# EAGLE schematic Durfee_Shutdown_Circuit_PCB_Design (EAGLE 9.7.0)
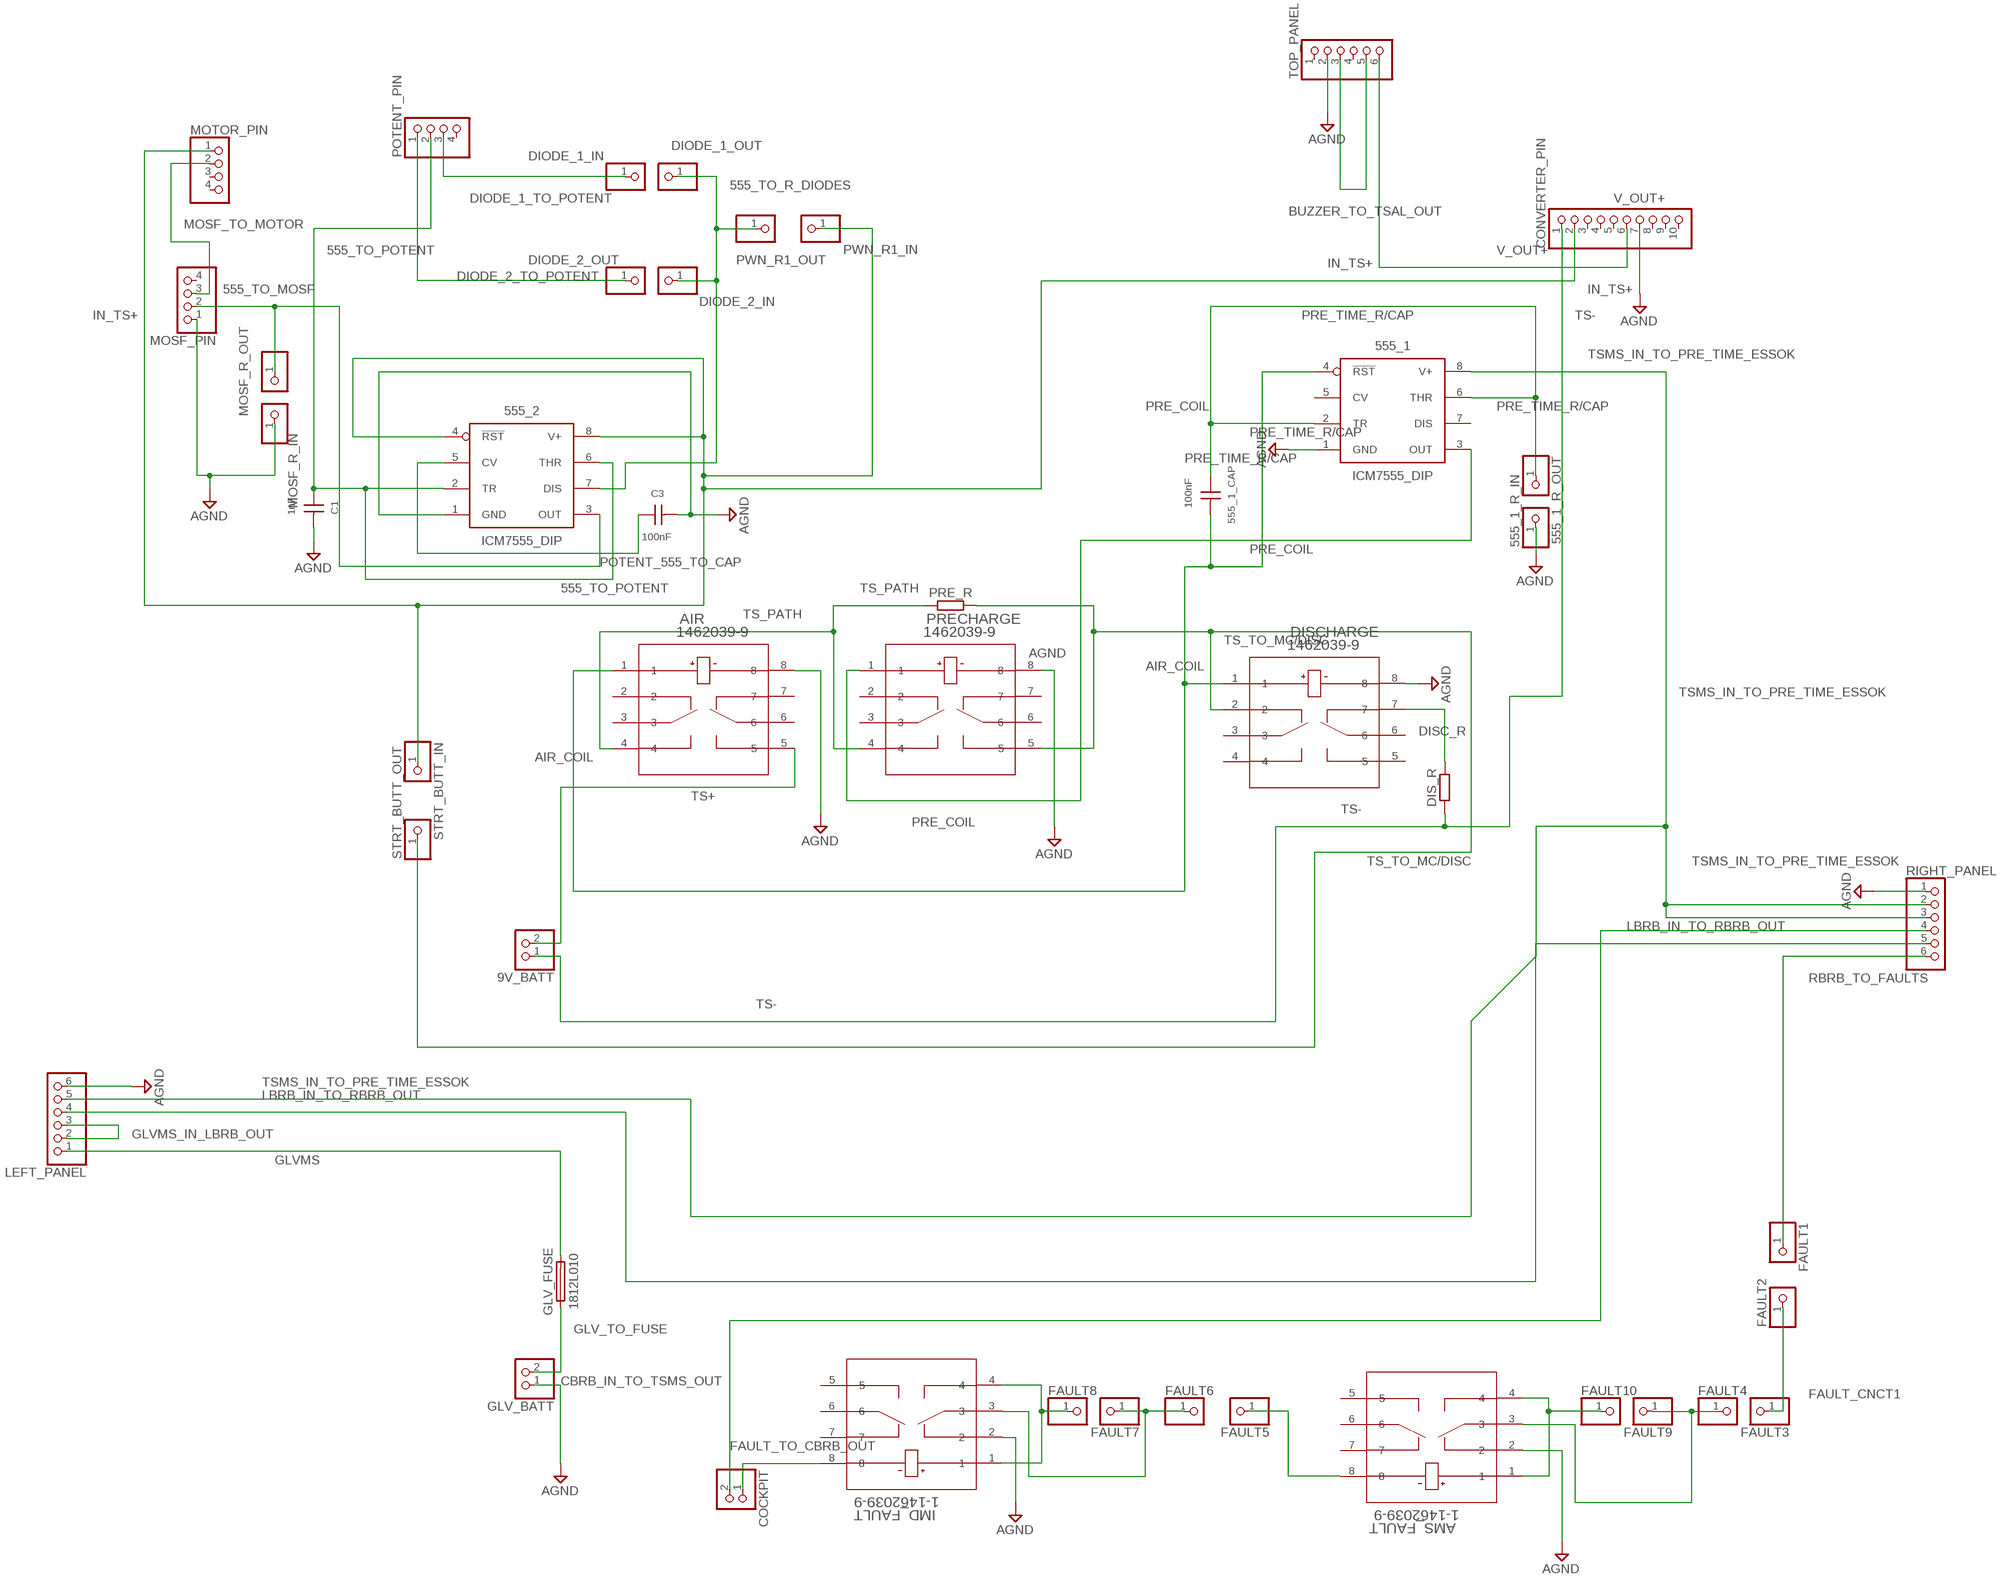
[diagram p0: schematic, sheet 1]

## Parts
9V_BATT  PINHD-1X2  [1X02]
555_1  ICM7555_DIP  [DIP826W53P254L959H508Q8B]
555_1_CAP  100nF  WCAP-CSGP_0603_885012206071_25V(DC)_R  [WCAP-CSGP_0603_R]
555_1_R_IN  PINHD-1X1  [1X01]
555_1_R_OUT  PINHD-1X1  [1X01]
555_2  ICM7555_DIP  [DIP826W53P254L959H508Q8B]
AIR  1462039-9  [RELAY8_SMTGUL]
AMS_FAULT  1-1462039-9  [RELAY8_SMTGUL]
C1  1nF  WCAP-CSGP_0402_885012205044_25V(DC)  [WCAP-CSGP_0402]
C3  100nF  WCAP-CSGP_0603_885012206071_25V(DC)_R  [WCAP-CSGP_0603_R]
COCKPIT  PINHD-1X2  [1X02]
CONVERTER_PIN  PINHD-1X10  [1X10]
DIODE_1_IN  PINHD-1X1  [1X01]
DIODE_1_OUT  PINHD-1X1  [1X01]
DIODE_2_IN  PINHD-1X1  [1X01]
DIODE_2_OUT  PINHD-1X1  [1X01]
DIS_R  R_AXIAL-7.2MM-PITCH  [RESAD724W46L381D178B]
DISCHARGE  1462039-9  [RELAY8_SMTGUL]
FAULT1  PINHD-1X1  [1X01]
FAULT2  PINHD-1X1  [1X01]
FAULT3  PINHD-1X1  [1X01]
FAULT4  PINHD-1X1  [1X01]
FAULT5  PINHD-1X1  [1X01]
FAULT6  PINHD-1X1  [1X01]
FAULT7  PINHD-1X1  [1X01]
FAULT8  PINHD-1X1  [1X01]
FAULT9  PINHD-1X1  [1X01]
FAULT10  PINHD-1X1  [1X01]
GLV_BATT  PINHD-1X2  [1X02]
GLV_FUSE  1812L010  [FUSC4532X125]
IMD_FAULT  1-1462039-9  [RELAY8_SMTGUL]
LEFT_PANEL  PINHD-1X6  [1X06]
MOSF_PIN  PINHD-1X4  [1X04]
MOSF_R_IN  PINHD-1X1  [1X01]
MOSF_R_OUT  PINHD-1X1  [1X01]
MOTOR_PIN  PINHD-1X4  [1X04]
POTENT_PIN  PINHD-1X4  [1X04]
PRE_R  R_AXIAL-7.2MM-PITCH  [RESAD724W46L381D178B]
PRECHARGE  1462039-9  [RELAY8_SMTGUL]
PWN_R1_IN  PINHD-1X1  [1X01]
PWN_R1_OUT  PINHD-1X1  [1X01]
RIGHT_PANEL  PINHD-1X6  [1X06]
STRT_BUTT_IN  PINHD-1X1  [1X01]
STRT_BUTT_OUT  PINHD-1X1  [1X01]
TOP_PANEL  PINHD-1X6  [1X06]

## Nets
555_TO_MOSF: 555_2.3(OUT) MOSF_PIN.2 MOSF_R_OUT.1
555_TO_POTENT: 555_2.2(TR) 555_2.6(THR) C1.1 POTENT_PIN.2
555_TO_R_DIODES: 555_2.7(DIS) DIODE_1_OUT.1 DIODE_2_IN.1 PWN_R1_OUT.1
AGND: 555_1.1(GND) 555_1_R_IN.1 555_2.1(GND) AIR.8 AMS_FAULT.2 C1.2 C3.2 CONVERTER_PIN.7 DISCHARGE.8 GLV_BATT.1 IMD_FAULT.2 LEFT_PANEL.6 MOSF_PIN.1 MOSF_R_IN.1 PRECHARGE.8 RIGHT_PANEL.1 TOP_PANEL.2
AIR_COIL: 555_1.4(!RST) 555_1_CAP.2 AIR.1 DISCHARGE.1
BUZZER_TO_TSAL_OUT: TOP_PANEL.3 TOP_PANEL.5
CBRB_IN_TO_TSMS_OUT: COCKPIT.2 RIGHT_PANEL.4
DIODE_1_TO_POTENT: DIODE_1_IN.1 POTENT_PIN.3
DIODE_2_TO_POTENT: DIODE_2_OUT.1 POTENT_PIN.1
DISC_R: DIS_R.2 DISCHARGE.7
FAULT_CNCT1: FAULT2.1 FAULT3.1
FAULT_TO_CBRB_OUT: COCKPIT.1 IMD_FAULT.8
GLV_TO_FUSE: GLV_BATT.2 GLV_FUSE.1
GLVMS: GLV_FUSE.2 LEFT_PANEL.1
GLVMS_IN_LBRB_OUT: LEFT_PANEL.2 LEFT_PANEL.3
IN_TS+: 555_2.4(!RST) 555_2.8(V+) CONVERTER_PIN.2 MOTOR_PIN.1 PWN_R1_IN.1 STRT_BUTT_IN.1
LBRB_IN_TO_RBRB_OUT: LEFT_PANEL.4 RIGHT_PANEL.5
MOSF_TO_MOTOR: MOSF_PIN.3 MOTOR_PIN.2
N$1: FAULT8.1 IMD_FAULT.1 IMD_FAULT.4
N$2: AMS_FAULT.3 FAULT4.1 FAULT9.1
N$3: FAULT6.1 FAULT7.1 IMD_FAULT.3
N$5: AMS_FAULT.8 FAULT5.1
N$6: AMS_FAULT.1 AMS_FAULT.4 FAULT10.1
POTENT_555_TO_CAP: 555_2.5(CV) C3.1
PRE_COIL: 555_1.3(OUT) PRECHARGE.1
PRE_TIME_R/CAP: 555_1.2(TR) 555_1.6(THR) 555_1_CAP.1 555_1_R_OUT.1
RBRB_TO_FAULTS: FAULT1.1 RIGHT_PANEL.6
TS+: 9V_BATT.2 AIR.5
TS-: 9V_BATT.1 CONVERTER_PIN.1 DIS_R.1
TS_PATH: AIR.4 PRE_R.1 PRECHARGE.4
TS_TO_MC/DISC: DISCHARGE.2 PRE_R.2 PRECHARGE.5 STRT_BUTT_OUT.1
TSMS_IN_TO_PRE_TIME_ESSOK: 555_1.8(V+) LEFT_PANEL.5 RIGHT_PANEL.2 RIGHT_PANEL.3
V_OUT+: CONVERTER_PIN.6 TOP_PANEL.6
Unconnected: 555_1.5(CV) 555_1.7(DIS) AIR.2 AIR.3 AIR.6 AIR.7 AMS_FAULT.5 AMS_FAULT.6 AMS_FAULT.7 CONVERTER_PIN.3 CONVERTER_PIN.4 CONVERTER_PIN.5 CONVERTER_PIN.8 CONVERTER_PIN.9 CONVERTER_PIN.10 DISCHARGE.3 DISCHARGE.4 DISCHARGE.5 DISCHARGE.6 IMD_FAULT.5 IMD_FAULT.6 IMD_FAULT.7 MOSF_PIN.4 MOTOR_PIN.3 MOTOR_PIN.4 POTENT_PIN.4 PRECHARGE.2 PRECHARGE.3 PRECHARGE.6 PRECHARGE.7 TOP_PANEL.1 TOP_PANEL.4

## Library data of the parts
9V_BATT COCKPIT GLV_BATT = pinhead:PINHD-1X2: PIN HEADER
555_1 555_2 = IC_Clock-Timing:*555: TIMER 555 General purpose precision timers NE555 : Texas Datasheet, Diodes Incorporated Datasheet LM555 Datasheet LMC555 Datasheet ICM7555 : Maxim Integrated Datasheet, Renesas Electronics America Inc Datasheet; CATEGORY: IC_Clock-Timing; CURRENT-SUPPLY: 60µA; DESCRIPTION: IC OSC SINGLE TIMER 1MHZ 8DIP; FREQUENCY: 1MHz; MANUFACTURER: Renesas Electronics America Inc; MPN: ICM7555IPAZ; OPERATING_TEMP: -25°C to 85°C; PART_STATUS: Active; ROHS_COMPLIANT: ROHS3 Compliant; SUB-CATEGORY: Timer
555_1_CAP C3 = Wurth_Capacitors_WCAP-CSGP:WCAP-CSGP_0603: WCAP-CSGP MLCCs 0603; CERAMIC-TYPE: X7R Class II; DATASHEET-URL: https://www.we-online.com/redexpert/spec/885012206071?ae; DF: 3.5%; HEIGHT: 0.8mm; MOUNT: SMT; OPERATING-TEMPERATURE: -55 up to +125 °C; PART-NUMBER: 885012206071; QMIN: -; RISO: 5GOhm; SIZE: 0603; TECHNICAL-REFERENCE: X7R0603104K025DFCT10000; VR: 25V(DC)
555_1_R_IN 555_1_R_OUT DIODE_1_IN DIODE_1_OUT DIODE_2_IN DIODE_2_OUT FAULT1-FAULT10 MOSF_R_IN MOSF_R_OUT PWN_R1_IN PWN_R1_OUT STRT_BUTT_IN STRT_BUTT_OUT = pinhead:PINHD-1X1: PIN HEADER
AIR DISCHARGE PRECHARGE = Relays:1462039-9; BUILT_BY: EMA_UL_Team; CATEGORY: Signal Relays; COPYRIGHT: Copyright (C) 2016 Accelerated Designs. All rights reserved; DESCRIPTION: IM48DGR=IM RELAY 100 MW 2.4 V; MANUFACTURER_PART_NUMBER: 1462039-9; PART_STATUS: active; SERIES: Axicom IM; VENDOR: TE Connectivity
AMS_FAULT IMD_FAULT = Relays:1-1462039-9; BUILT_BY: EMA_UL_Team; CATEGORY: Signal Relays; CONTACT_ARRANGEMENT: 2 Form C (CO); COPYRIGHT: Copyright (C) 2016 Accelerated Designs. All rights reserved; DESCRIPTION: IM42DGR=IM RELAY 100 MW 4.5 V; MANUFACTURER_PART_NUMBER: 1-1462039-9; MAXIMUM_SWITCHING_CURRENT: -; MAXIMUM_SWITCHING_VOLTAGE: -; PART_STATUS: active; PRODUCT_TYPE: Relay; RELAY_TYPE: IM Relay; SERIES: Axicom IM; TE_PART_NUMBER: 1-1462039-9; VENDOR: TE Connectivity
C1 = Wurth_Capacitors_WCAP-CSGP:WCAP-CSGP_0402: WCAP-CSGP MLCCs 0402; CERAMIC-TYPE: X7R Class II; DATASHEET-URL: https://www.we-online.com/redexpert/spec/885012205044?ae; DF: 3.5%; HEIGHT: 0.5mm; MOUNT: SMT; OPERATING-TEMPERATURE: -55 up to +125 °C; PART-NUMBER: 885012205044; QMIN: -; RISO: 10GOhm; SIZE: 0402; TECHNICAL-REFERENCE: X7R0402102K025DFCT10000; VR: 25V(DC)
CONVERTER_PIN = pinhead:PINHD-1X10: PIN HEADER
DIS_R PRE_R = Resistor:R: Resistor Fixed - Generic; CATEGORY: Resistor; SUB-CATEGORY: Fixed
GLV_FUSE = Fuse:1812L: 1812L Series PTC provides surface mount overcurrent; CATEGORY: FUSE; DESCRIPTION: Resettable PTCs; MANUFACTURER: Littlefuse; MPN: 1812L010; OPERATING_TEMPERATURE: -40°C to +85°C; PART_STATUS: ACTIVE; ROHS_COMPLIANCE: RoHS Compliant; SERIES: 1812L; SUBCATEGORY: Resettable; TYPE: PTC
LEFT_PANEL RIGHT_PANEL TOP_PANEL = pinhead:PINHD-1X6: PIN HEADER
MOSF_PIN MOTOR_PIN POTENT_PIN = pinhead:PINHD-1X4: PIN HEADER

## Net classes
0 default: width 0.953 mm

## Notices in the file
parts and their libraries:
Wurth_Capacitors_WCAP-CSGP: Copyright: Würth Elektronik
